(* Logix 5000 AddOnInstructionDefinition export Gate_Flop; software revision 20.01 *)

TYPE Gate_Flop_Type :   // Flop Gate data
STRUCT
   Run_Status : BOOL;   // Run Status (1=running)
   Left_Status : BOOL;   // Left LS status (1=left position)
   Right_Status : BOOL;   // Right LS status (1=right position)
   Any_Fail : BOOL;   // Overall Failure Alarm (1= alarm)
   HOA_Fail : BOOL;   // HOA-switch-not-in-auto alarm (1-alarm)
   FTL_Fail : BOOL;   // Fail-to-divert-left failure alarm (1=alarm)
   FTR_Fail : BOOL;   // Fail-to-divert-right failure alarm (1=alarm)
   Seq_Left : BOOL;   // Gate open initiated from sequence
   Seq_Right : BOOL;   // Gate close initiated from sequence
END_STRUCT
END_TYPE

ADD_ON_INSTRUCTION Gate_Flop   (* revision 1.3 *)
// Flop gate control
// Revision note:
// Use CMP for device number
VAR_INPUT
   Left_LS : BOOL; {required}   // Gate-left limit switch physical input
   Right_LS : BOOL; {required}   // Gate-right limit switch physical input
   HOA_Switch : BOOL; {required}   // Hand-Off-Auto switch contact physical input (on when in Auto position)
   Alarm_Reset : BOOL; {required}   // Resets alarms
   Maint : BOOL; {required}   // Unit Maintenance/Operate Privilege
   Man_Left : BOOL; {required}   // Manual left for unit
   Man_Right : BOOL; {required}   // Manual right for unit
   Select_Dev_Num : DINT; {required}   // Number of device started/stopped at OI
   This_Dev_Num : DINT; {required}   // Number of this device for OI control
END_VAR
VAR_OUTPUT
   Sol_Left : BOOL; {access Read Only, required}   // Left position physical output
   Sol_Right : BOOL; {access Read Only, required}   // Right position physical output
END_VAR
VAR_IN_OUT
   Tag : Gate_Flop_Type; {required}   // Flop Gate Tag
END_VAR
VAR
   Left_Req : BOOL;   // Internal used for left logic
   Right_Req : BOOL;   // Internal used for right logic
   Fail_Tmr : TIMER := (PRE := 20000);   // Timer for alarms
END_VAR

ROUTINE Logic   (* ladder *)
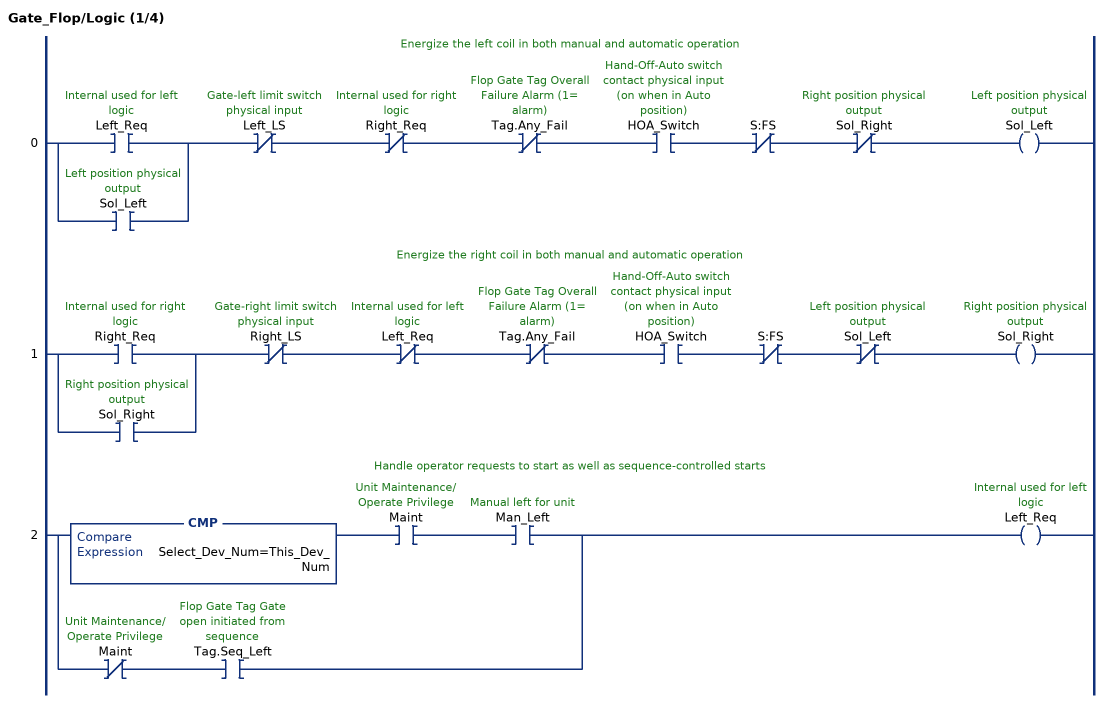
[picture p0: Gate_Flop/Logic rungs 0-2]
   // Energize the left coil in both manual and automatic operation
   0: [XIC(Left_Req) ,XIC(Sol_Left) ]XIO(Left_LS)XIO(Right_Req)XIO(Tag.Any_Fail)XIC(HOA_Switch)XIO(S:FS)XIO(Sol_Right)OTE(Sol_Left);
   // Energize the right coil in both manual and automatic operation
   1: [XIC(Right_Req) ,XIC(Sol_Right) ]XIO(Right_LS)XIO(Left_Req)XIO(Tag.Any_Fail)XIC(HOA_Switch)XIO(S:FS)XIO(Sol_Left)OTE(Sol_Right);
   // Handle operator requests to start as well as sequence-controlled starts
   2: [CMP(Select_Dev_Num=This_Dev_Num) XIC(Maint) XIC(Man_Left) ,XIO(Maint) XIC(Tag.Seq_Left) ]OTE(Left_Req);
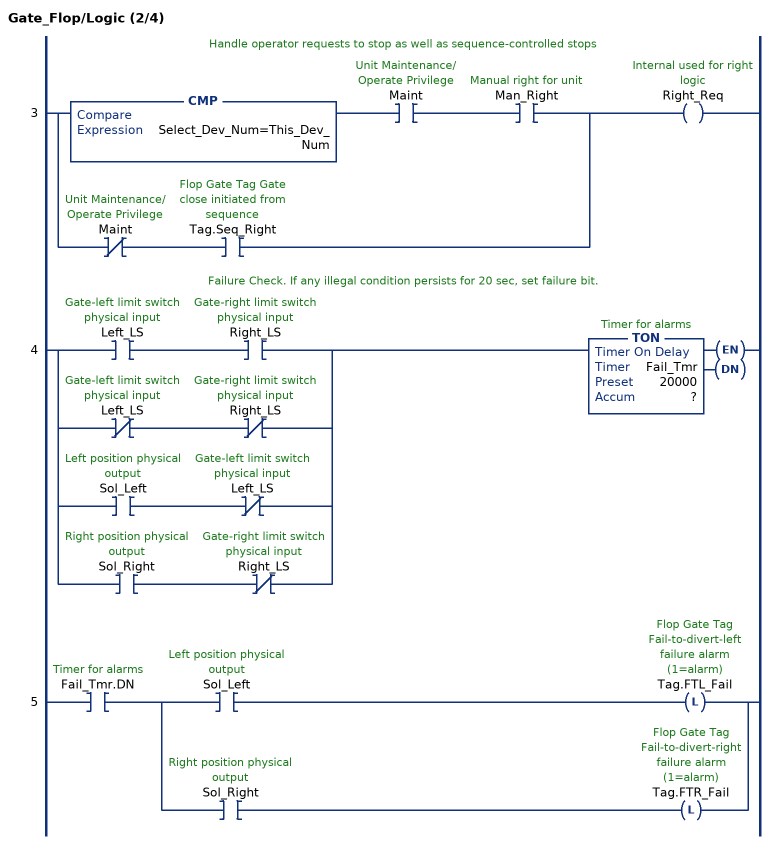
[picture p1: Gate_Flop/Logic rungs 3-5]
   // Handle operator requests to stop as well as sequence-controlled stops
   3: [CMP(Select_Dev_Num=This_Dev_Num) XIC(Maint) XIC(Man_Right) ,XIO(Maint) XIC(Tag.Seq_Right) ]OTE(Right_Req);
   // Failure Check. If any illegal condition persists for 20 sec, set failure bit.
   4: [XIC(Left_LS) XIC(Right_LS) ,XIO(Left_LS) XIO(Right_LS) ,XIC(Sol_Left) XIO(Left_LS) ,XIC(Sol_Right) XIO(Right_LS) ]TON(Fail_Tmr,?,?);
   5: XIC(Fail_Tmr.DN)[XIC(Sol_Left) OTL(Tag.FTL_Fail) ,XIC(Sol_Right) OTL(Tag.FTR_Fail) ];
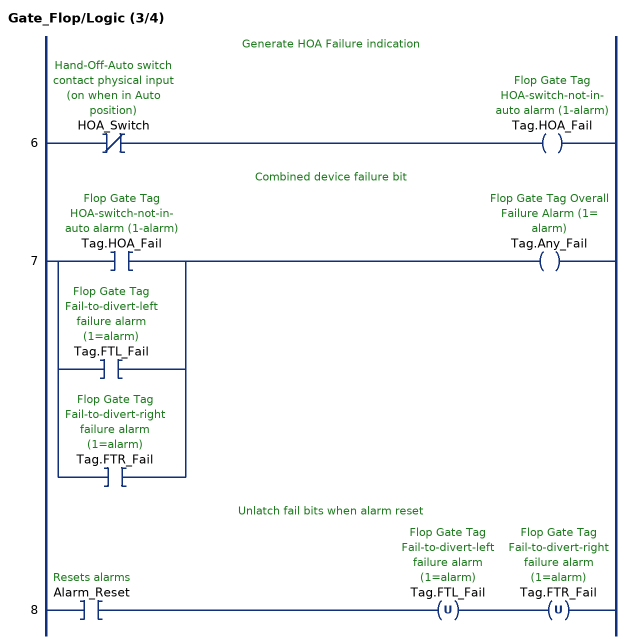
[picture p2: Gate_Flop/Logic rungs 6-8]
   // Generate HOA Failure indication
   6: XIO(HOA_Switch)OTE(Tag.HOA_Fail);
   // Combined device failure bit
   7: [XIC(Tag.HOA_Fail) ,XIC(Tag.FTL_Fail) ,XIC(Tag.FTR_Fail) ]OTE(Tag.Any_Fail);
   // Unlatch fail bits when alarm reset
   8: XIC(Alarm_Reset)OTU(Tag.FTL_Fail)OTU(Tag.FTR_Fail);
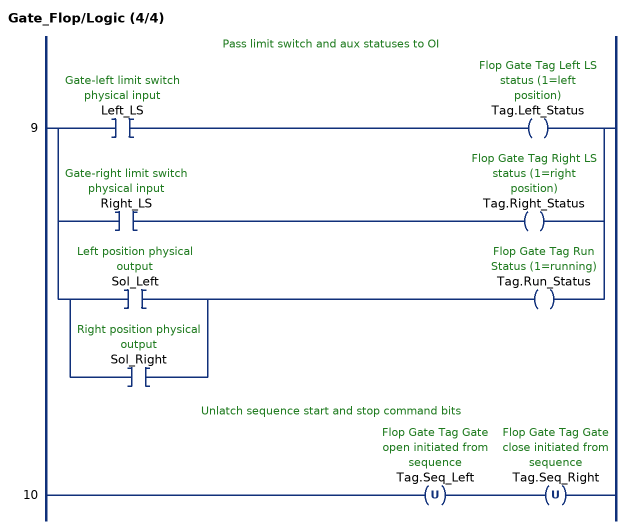
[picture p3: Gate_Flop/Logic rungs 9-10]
   // Pass limit switch and aux statuses to OI
   9: [XIC(Left_LS) OTE(Tag.Left_Status) ,XIC(Right_LS) OTE(Tag.Right_Status) ,[XIC(Sol_Left) ,XIC(Sol_Right) ] OTE(Tag.Run_Status) ];
   // Unlatch sequence start and stop command bits
   10: OTU(Tag.Seq_Left)OTU(Tag.Seq_Right);
END_ROUTINE
END_ADD_ON_INSTRUCTION
